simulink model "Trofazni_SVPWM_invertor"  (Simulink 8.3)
settings: Solver=ode3  StartTime=0.0  StopTime=Tfinal  FixedStep=Tsim  MaxStep=1e-7  RelTol=1e-3
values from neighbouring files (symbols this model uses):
  fdq = 50    [Trofazni_SVPWM_invertor_parametri.m]
  fpwm = 20000    [Trofazni_SVPWM_invertor_parametri.m]
  L = 76e-3    (= 0.076)    [Trofazni_SVPWM_invertor_parametri.m]
  MOD = TROUGAO    (= 1)    [Trofazni_SVPWM_invertor_parametri.m]
  R = 10.0    (= 10)    [Trofazni_SVPWM_invertor_parametri.m]
  Tdt = 1e-6    (= 1e-06)    [Trofazni_SVPWM_invertor_parametri.m]
  Tpwm = 1/fpwm    (= 5e-05)    [Trofazni_SVPWM_invertor_parametri.m]
  ugao_dq = 45    [Trofazni_SVPWM_invertor_parametri.m]
  Vd = 200    [Trofazni_SVPWM_invertor_parametri.m]
  Vdc = sqrt(2)*400    [Trofazni_SVPWM_invertor_parametri.m]
  Vq = 0    [Trofazni_SVPWM_invertor_parametri.m]
undefined symbols (not defined in the file or in its folder): bin2dec
libraries: powerlib x18, simulink x3, simulink_extras x1

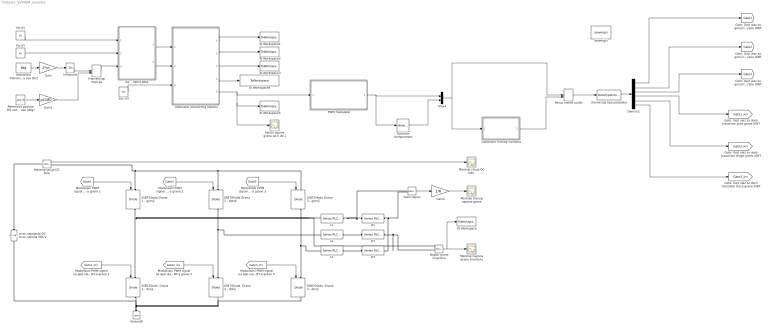
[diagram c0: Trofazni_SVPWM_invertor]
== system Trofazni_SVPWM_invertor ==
  Demux2 : Demux  Outputs=6
  Faktor ispune grana od 0 do 1 : Scope
  Fazni napon : powerlib/Measurements/Voltage Measurement  PhasorSimulation=off  OutputType=Complex  PSBequivalent=0
  Frekvencija/ Pozicija : ManualSwitch
  Gain : Gain  Gain=2*pi
  Gain1 : Gain  Gain=pi/180
  Gain2 : Gain  Gain=1/R
  Generator mrtvog vremena : Subsystem
  Ground9 : powerlib/Elements/Ground  LConnTagsString=a
  IGBT/Dioda Grana 1 - gornji : powerlib/Power Electronics/IGBT//Diode  Ron=Ron  Rs=Rsnub  Cs=inf  Measurements=on
  IGBT/Dioda Grana 2 - gornji : powerlib/Power Electronics/IGBT//Diode  Ron=Ron  Rs=Rsnub  Cs=inf  Measurements=on
  IGBT/Dioda Grana 3 - gornji : powerlib/Power Electronics/IGBT//Diode  Ron=Ron  Rs=Rsnub  Cs=inf  Measurements=on
  IGBT/Dioda  Grana 1 - donji : powerlib/Power Electronics/IGBT//Diode  Ron=Ron  Rs=Rsnub  Cs=inf  Measurements=on
  IGBT/Dioda  Grana 2 - donji : powerlib/Power Electronics/IGBT//Diode  Ron=Ron  Rs=Rsnub  Cs=inf  Measurements=on
  IGBT/Dioda  Grana 3 - donji : powerlib/Power Electronics/IGBT//Diode  Ron=Ron  Rs=Rsnub  Cs=inf  Measurements=on
  Integrator : Integrator
  Izvor napajanja DC izvor napona 565 V : powerlib/Electrical Sources/DC Voltage Source  Amplitude=Vdc  Measurements=None
  Konverzija tipa podataka : DataTypeConversion
  L1 : powerlib/Elements/Series RLC Branch  LConnTagsString=__new0  RConnTagsString=__new0  BranchType=L  Resistance=1  Inductance=L  SetiL0=off  InitialCurrent=0  Capacitance=0  Setx0=off  InitialVoltage=0  Measurements=None
  L2 : powerlib/Elements/Series RLC Branch  LConnTagsString=__new0  RConnTagsString=__new0  BranchType=L  Resistance=1  Inductance=L  SetiL0=off  InitialCurrent=0  Capacitance=0  Setx0=off  InitialVoltage=0  Measurements=None
  L3 : powerlib/Elements/Series RLC Branch  LConnTagsString=__new0  RConnTagsString=__new0  BranchType=L  Resistance=1  Inductance=L  SetiL0=off  InitialCurrent=0  Capacitance=0  Setx0=off  InitialVoltage=0  Measurements=None
  Merenje faznog napona grane : Scope
  Merenje napona grane invertora : Scope
  Merenje struje DC kola : powerlib/Measurements/Current Measurement  PhasorSimulation=off  OutputType=Complex  PSBequivalent=0
  "Merenje struje DC kola " : Scope
  Modulator prostornog vektora : Subsystem
  Mrtvo vreme on/off : ManualSwitch
  Mux4 : Mux  Inputs=2
  Napon grane invertora : powerlib/Measurements/Voltage Measurement  PhasorSimulation=off  OutputType=Complex  PSBequivalent=0
  Operator Komplement : simulink/Logic and Bit Operations/Bitwise Operator  logicop=NOT  UseBitMask=off  BitMask=bin2dec('11011001')  BitMaskRealWorld=Stored Integer
  PWM modulator : Subsystem
  R1 : powerlib/Elements/Series RLC Branch  LConnTagsString=__new0  RConnTagsString=__new0  BranchType=R  Resistance=R  Inductance=1e-3  SetiL0=off  InitialCurrent=0  Capacitance=0  Setx0=off  InitialVoltage=0  Measurements=None
  R2 : powerlib/Elements/Series RLC Branch  LConnTagsString=__new0  RConnTagsString=__new0  BranchType=R  Resistance=R  Inductance=1e-3  SetiL0=off  InitialCurrent=0  Capacitance=0  Setx0=off  InitialVoltage=0  Measurements=None
  R3 : powerlib/Elements/Series RLC Branch  LConnTagsString=__new0  RConnTagsString=__new0  BranchType=R  Resistance=R  Inductance=1e-3  SetiL0=off  InitialCurrent=0  Capacitance=0  Setx0=off  InitialVoltage=0  Measurements=None
  Referenca frekvencije DQ sistema osa [Hz] : Constant  Value=fdq
  Referenca pozicije DQ sistema osa [deg] : Constant  Value=ugao_dq
  To Workspace : ToWorkspace  VariableName=Vout  SampleTime=-1
  To Workspace1 : ToWorkspace  VariableName=ugao  SampleTime=-1
  To Workspace2 : ToWorkspace  VariableName=BrojSektora  SampleTime=-1
  To Workspace3 : ToWorkspace  VariableName=T1T2T0  SampleTime=-1
  To Workspace4 : ToWorkspace  VariableName=LONG_MIDDLE_SHORT  SampleTime=-1
  To Workspace5 : ToWorkspace  VariableName=Tabc  SampleTime=-1
  Vd (V) : Constant  Value=Vd
  Vdc (V) : Constant  Value=Vdc
  Vq (V) : Constant  Value=Vq
  dq  - alpha beta- : Subsystem
  powergui : powerlib/powergui  Priority=1  SimulationMode=Continuous  SolverType=Tustin  SampleTime=50e-6  frequency=60  SPID=on  DisableSnubberDevices=off  DisableRonSwitches=off  DisableVfSwitches=off  SwTol=0  Interpol=off  DisplayEquations=off  Ts=0  methode=off  frequencyindice=0  Pbase=100e6  ErrMax=1e-4  Iterations=50  UnitsV=kV  UnitsW=MW  FunctionMessages=off  echomessages=off  HookPort=off  EnableUseOfTLC=off  x0status=blocks  RestoreLinks=warning  ResistiveCurrentMeasurement=off  Frange=[0:2:500]  Ylog=off  Xlog=on  ShowGrid=off  save=off  variable=ZData  structure=TABC  ZoomFFT=on  StartTime=0.05  cycles=1  DisplayStyle=2  fundamental=50  FreqAxis=off  MaxFrequency=1000  frequencyindicesteady=1  RmsSteady=1  display=off
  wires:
  Napon grane invertora/1 -> To Workspace/1, Merenje napona grane invertora/1
  [Gate1] -> IGBT/Dioda Grana 1 - gornji/1
  [Gate1_inv] -> IGBT/Dioda  Grana 1 - donji/1
  [Gate2] -> IGBT/Dioda Grana 2 - gornji/1
  [Gate2_inv] -> IGBT/Dioda  Grana 2 - donji/1
  [Gate3] -> IGBT/Dioda Grana 3 - gornji/1
  [Gate3_inv] -> IGBT/Dioda  Grana 3 - donji/1
  PWM modulator/1(Modulisani PWM signal) -> Operator Komplement/1, Mux4/1
  Vq (V)/1 -> dq  - alpha beta-/2(Vq_ref)
  Gain/1 -> Integrator/1
  Referenca frekvencije DQ sistema osa [Hz]/1 -> Gain/1
  dq  - alpha beta-/1(Valpha_ref) -> Modulator prostornog vektora/1(Valpha)
  dq  - alpha beta-/2(Vbeta_ref) -> Modulator prostornog vektora/2(Vbeta)
  Modulator prostornog vektora/1(ugao dq) -> To Workspace1/1
  Modulator prostornog vektora/2(Broj sektora) -> To Workspace2/1
  Modulator prostornog vektora/3(T1T2T0) -> To Workspace3/1
  Vdc (V)/1 -> Modulator prostornog vektora/3(Vdc)
  Modulator prostornog vektora/4(LONG_MIDDLE_SHORT) -> To Workspace4/1
  Integrator/1 -> Frekvencija/ Pozicija/1
  Referenca pozicije DQ sistema osa [deg]/1 -> Gain1/1
  Gain1/1 -> Frekvencija/ Pozicija/2
  Frekvencija/ Pozicija/1 -> dq  - alpha beta-/3(ugao)
  Vd (V)/1 -> dq  - alpha beta-/1(Vd_ref)
  Modulator prostornog vektora/5(Tabc) -> PWM modulator/1(Faktor ispune), Faktor ispune grana od 0 do 1/1, To Workspace5/1
  Merenje struje DC kola/1 -> "Merenje struje DC kola "/1
  Fazni napon/1 -> Gain2/1
  Gain2/1 -> Merenje faznog napona grane/1
  Operator Komplement/1 -> Mux4/2
  Mux4/1 -> Mrtvo vreme on/off/1, Generator mrtvog vremena/1(Ton)
  Demux2/4 -> [Gate1_inv]
  Demux2/5 -> [Gate2_inv]
  Demux2/6 -> [Gate3_inv]
  Demux2/1 -> [Gate1]
  Demux2/2 -> [Gate2]
  Demux2/3 -> [Gate3]
  Mrtvo vreme on/off/1 -> Konverzija tipa podataka/1
  Generator mrtvog vremena/1(Ton dt) -> Mrtvo vreme on/off/2
  Konverzija tipa podataka/1 -> Demux2/1
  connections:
  IGBT/Dioda Grana 2 - gornji/LConn1 -- Merenje struje DC kola/RConn1 -- IGBT/Dioda Grana 1 - gornji/LConn1 -- IGBT/Dioda Grana 3 - gornji/LConn1
  Ground9/LConn1 -- Izvor napajanja DC izvor napona 565 V/LConn1 -- IGBT/Dioda  Grana 3 - donji/RConn1 -- IGBT/Dioda  Grana 2 - donji/RConn1 -- IGBT/Dioda  Grana 1 - donji/RConn1
  IGBT/Dioda Grana 1 - gornji/RConn1 -- L1/LConn1 -- Napon grane invertora/LConn1 -- IGBT/Dioda  Grana 1 - donji/LConn1
  IGBT/Dioda Grana 2 - gornji/RConn1 -- L2/LConn1 -- IGBT/Dioda  Grana 2 - donji/LConn1
  IGBT/Dioda Grana 3 - gornji/RConn1 -- L3/LConn1 -- IGBT/Dioda  Grana 3 - donji/LConn1
  L1/RConn1 -- Fazni napon/LConn1 -- R1/LConn1
  L2/RConn1 -- R2/LConn1
  L3/RConn1 -- R3/LConn1
  Izvor napajanja DC izvor napona 565 V/RConn1 -- Merenje struje DC kola/LConn1
  R2/RConn1 -- Napon grane invertora/LConn2 -- R3/RConn1 -- R1/RConn1 -- Fazni napon/LConn2

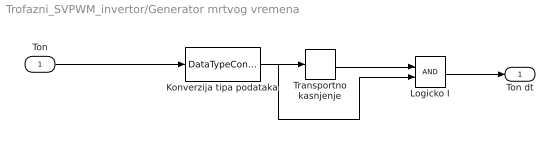
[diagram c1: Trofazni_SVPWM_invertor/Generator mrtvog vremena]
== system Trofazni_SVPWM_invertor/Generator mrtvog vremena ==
  Ton : Inport
  Konverzija tipa podataka : DataTypeConversion
  Logicko I : Logic  AllPortsSameDT=off  OutDataTypeStr=boolean
  Transportno kasnjenje : TransportDelay  DelayTime=Tdt
  Ton dt : Outport
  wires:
  Transportno kasnjenje/1 -> Logicko I/1
  Logicko I/1 -> Ton dt/1
  Ton/1 -> Konverzija tipa podataka/1
  Konverzija tipa podataka/1 -> Logicko I/2, Transportno kasnjenje/1

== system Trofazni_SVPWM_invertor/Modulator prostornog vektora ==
  note: Deo za izraunavanje trajanja aktivnih i nultih vektora
  note: Dodela vremena provoenaj fazama u zavisnosti od broja sektora
  Valpha : Inport
  Vbeta : Inport  Port=2
  Vdc : Inport  Port=3
  Ako je T0 < 0  SATURACIJA : Switch
  Blok - Broj sektora : Subsystem
  Gain2 : Gain  Gain=2*fpwm
  LONG : Fcn  Expr=u(3)/2+u(1)+u(2)
  MIDDLE : Fcn  Expr=u(3)/2+u(2)
  MIDDLE1 : Fcn  Expr=u(3)/2+u(1)
  Mux{1..2,5..11} (9 alike) : Mux  Inputs=3
  Mux3 : Mux  Inputs=2
  Mux4 : Mux  Inputs=2
  SHORT : Fcn  Expr=u(3)/2
  Saturacija : Saturate  UpperLimit=6  LowerLimit=0
  T0 kalulator : Fcn  Expr=Tpwm/2-u(1)-u(2)
  Tk kalkulator : Fcn  Expr=(sqrt(3)/u(4))*(Tpwm/2)* (u(2)* sin(u(1)*pi/3)- u(3)*cos(u(1)*pi/3))
  Tk saturisano : Fcn  Expr=(Tpwm/2) *u(1)/(u(1)+u(2))
  Tk+1 kalkulator : Fcn  Expr=(sqrt(3)/u(4))*(Tpwm/2)* (-u(2)* sin((u(1)-1)*pi/3) + u(3)*cos((u(1)-1)*pi/3))
  Tk+1 saturisano : Fcn  Expr=(Tpwm/2) *u(2)/(u(1)+u(2))
  To Workspace : ToWorkspace  VariableName=Valpha_beta  SampleTime=-1
  U saturaciji T0=0 : Constant  Value=0
  Višeportni prekidac : MultiPortSwitch  Inputs=6
  ugao dq : Outport
  Broj sektora : Outport  Port=2
  T1T2T0 : Outport  Port=3
  LONG_MIDDLE_SHORT : Outport  Port=4
  Tabc : Outport  Port=5
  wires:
  Vbeta/1 -> Mux4/2
  Mux4/1 -> To Workspace/1, Blok - Broj sektora/1(V_alpha_beta), Mux1/2
  Valpha/1 -> Mux4/1
  Vdc/1 -> Mux1/3
  Blok - Broj sektora/2(Broj sektora) -> Broj sektora/1, Saturacija/1, Mux1/1
  Blok - Broj sektora/1(Ugao dq) -> ugao dq/1
  Mux1/1 -> Tk kalkulator/1, Tk+1 kalkulator/1
  Tk kalkulator/1 -> Mux2/1, Mux3/1
  Tk+1 kalkulator/1 -> Mux2/2, Mux3/2
  Mux2/1 -> Ako je T0 < 0  SATURACIJA/1
  Mux3/1 -> T0 kalulator/1, Tk saturisano/1, Tk+1 saturisano/1
  T0 kalulator/1 -> Mux2/3, Ako je T0 < 0  SATURACIJA/2
  LONG/1 -> Mux5/1, Mux6/2, Mux7/2, Mux8/3, Mux9/3, Mux10/1
  MIDDLE/1 -> Mux5/2, Mux7/3, Mux9/1
  SHORT/1 -> Mux5/3, Mux6/3, Mux7/1, Mux8/1, Mux9/2, Mux10/2
  Mux5/1 -> LONG_MIDDLE_SHORT/1, Višeportni prekidac/2
  Mux6/1 -> [Sec2_MLS]
  Mux7/1 -> [Sec3_SLM]
  Mux8/1 -> [Sec4_SML]
  Mux9/1 -> [Sec5_MSL]
  Mux10/1 -> [Sec6_LSM]
  [Sec2_MLS] -> Višeportni prekidac/3
  [Sec3_SLM] -> Višeportni prekidac/4
  [Sec4_SML] -> Višeportni prekidac/5
  [Sec5_MSL] -> Višeportni prekidac/6
  [Sec6_LSM] -> Višeportni prekidac/7
  Višeportni prekidac/1 -> Gain2/1
  Saturacija/1 -> Višeportni prekidac/1
  MIDDLE1/1 -> Mux6/1, Mux8/2, Mux10/3
  Tk+1 saturisano/1 -> Mux11/2
  Tk saturisano/1 -> Mux11/1
  Mux11/1 -> Ako je T0 < 0  SATURACIJA/3
  Ako je T0 < 0  SATURACIJA/1 -> T1T2T0/1, LONG/1, MIDDLE/1, SHORT/1, MIDDLE1/1
  U saturaciji T0=0/1 -> Mux11/3
  Gain2/1 -> Tabc/1

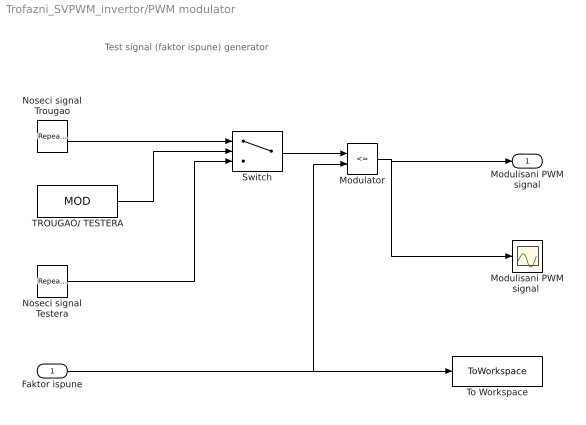
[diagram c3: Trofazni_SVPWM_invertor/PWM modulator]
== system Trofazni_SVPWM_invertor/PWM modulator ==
  note: Test signal (faktor ispune) generator
  Faktor ispune : Inport
  Modulator : RelationalOperator  Operator=<=  OutDataTypeStr=boolean
  "Modulisani PWM signal " : Scope
  Noseci signal Testera : simulink/Sources/Repeating Sequence  rep_seq_t=[0 Tpwm]  rep_seq_y=[0 1]
  Noseci signal Trougao : simulink/Sources/Repeating Sequence  rep_seq_t=[0 Tpwm/2 Tpwm]  rep_seq_y=[0 1 0]
  Switch : Switch  Criteria=u2 > Threshold
  TROUGAO/ TESTERA : Constant  Value=MOD
  To Workspace : ToWorkspace  VariableName=Upravljacka_prom  SampleTime=-1
  Modulisani PWM signal : Outport
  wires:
  Modulator/1 -> "Modulisani PWM signal "/1, Modulisani PWM signal/1
  Faktor ispune/1 -> To Workspace/1, Modulator/2
  Switch/1 -> Modulator/1
  Noseci signal Trougao/1 -> Switch/1
  Noseci signal Testera/1 -> Switch/3
  TROUGAO/ TESTERA/1 -> Switch/2

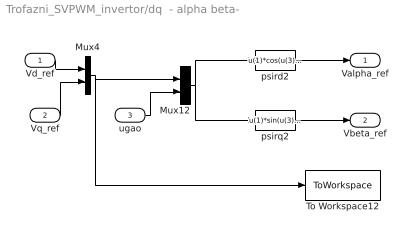
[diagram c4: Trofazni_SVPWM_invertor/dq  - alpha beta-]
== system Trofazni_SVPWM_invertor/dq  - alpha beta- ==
  Vd_ref : Inport
  Vq_ref : Inport  Port=2
  ugao : Inport  Port=3
  Mux12 : Mux  Inputs=2
  Mux4 : Mux  Inputs=2
  To Workspace12 : ToWorkspace  VariableName=Vdq  SampleTime=-1
  psird2 : Fcn  Expr=u(1)*cos(u(3))-u(2)*sin(u(3))
  psirq2 : Fcn  Expr=u(1)*sin(u(3))+u(2)*cos(u(3))
  Valpha_ref : Outport
  Vbeta_ref : Outport  Port=2
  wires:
  psirq2/1 -> Vbeta_ref/1
  Mux12/1 -> psird2/1, psirq2/1
  psird2/1 -> Valpha_ref/1
  ugao/1 -> Mux12/2
  Vd_ref/1 -> Mux4/1
  Mux4/1 -> Mux12/1, To Workspace12/1
  Vq_ref/1 -> Mux4/2

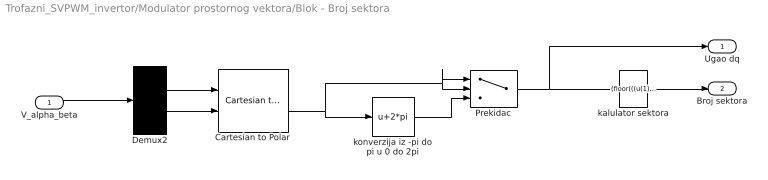
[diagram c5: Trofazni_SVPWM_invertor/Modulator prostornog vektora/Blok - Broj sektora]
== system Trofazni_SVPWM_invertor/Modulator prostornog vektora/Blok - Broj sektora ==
  V_alpha_beta : Inport
  Cartesian to Polar : simulink_extras/Transformations/Cartesian to Polar
  Demux2 : Demux  Outputs=2
  Prekidac : Switch
  kalulator sektora : Fcn  Expr=(floor(((u(1))/(2*pi))*6))+1
  konverzija iz -pi do pi u 0 do 2pi : Fcn  Expr=u+2*pi
  Ugao dq : Outport
  Broj sektora : Outport  Port=2
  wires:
  Cartesian to Polar/2 -> konverzija iz -pi do pi u 0 do 2pi/1, Prekidac/2, Prekidac/1
  konverzija iz -pi do pi u 0 do 2pi/1 -> Prekidac/3
  Prekidac/1 -> kalulator sektora/1, Ugao dq/1
  kalulator sektora/1 -> Broj sektora/1
  V_alpha_beta/1 -> Demux2/1
  Demux2/1 -> Cartesian to Polar/1
  Demux2/2 -> Cartesian to Polar/2
